(* Logix 5000 AddOnInstructionDefinition export AKD_Shutdown; software revision 26.01 *)

TYPE AKD_Status :   // All connections to the drive ethernet module are established and data is successfully transferring.
STRUCT
   Profile_In_Progress : BOOL;   // Profile Move In Progress
   Block_In_Execution : BOOL;   // Block In Execution
   On_Target_Position : BOOL;   // On Target Position (1=Current Position Equals Last Target Position)
   General_Fault : BOOL;   // General Fault
   Current_Direction : BOOL;   // Current Motor Direction (0=Reverse, 1=Forward)
   Home_Level : BOOL;   // Level of Home Input
   Reg_Level : BOOL;   // Level of Registration Input
   Enable : BOOL;   // State of Enable Output
   Fault_Input_Fault : BOOL;   // Fault Input Active
   Fwd_Limit : BOOL;   // Forward Input Active
   Rev_Limit : BOOL;   // Reverse Input Active
   Positive_Limit : BOOL;   // Positive Software Limit Exceeded
   Negative_Limit : BOOL;   // Negative Software Limit Exceeded
   FE_Fault : BOOL;   // Following Error Fault
   Block_Fault : BOOL;   // Block Execution Fault
   Load_Complete : BOOL;   // Command Message Successfully Loaded
END_STRUCT
END_TYPE

TYPE AKD_Control :   // Send Explicit Message
STRUCT
   Load_Data_Start_Profile : BOOL;   // Load Command Data / Start Profile Move
   Start_Block : BOOL;   // Execute Command block or block chain
   Incremental : BOOL;   // Incremental Position (0=Absolute, 1=Incremental)
   Direction : BOOL;   // Direction in Velocity Mode (0=Reverse, 1=Forward)
   Smooth_Stop : BOOL;   // Smooth / Controlled Stop w/ Deceleration
   Hard_Stop : BOOL;   // Hard / Immediate Stop
   Reg_Arm : BOOL;   // Arm the Registration Input
   Enable : BOOL;   // Enable Output
END_STRUCT
END_TYPE

TYPE AKD_Axis :   // Axis Data:
STRUCT
   Control : AKD_Control;   // Control bits to send to the drive
   Status : AKD_Status;   // Status bits received from the drive
   Input : AB:ETHERNET_MODULE_SINT_64Bytes:I:0;   // Data from the drive
   Output : AB:ETHERNET_MODULE_SINT_64Bytes:O:0;   // Data to the drive
   ResponseMsgType : SINT;   // Response type contained in latest IO response from drive. Used to check for errors
   CommandTimeout : INT;   // Time to allow for command response from drive. Dependent on scan rate and communicaiton rate
   PositionFeedback : DINT;   // Actual Position Value
   VelocityFeedback : DINT;   // Actual Velocity Value
END_STRUCT
END_TYPE

ADD_ON_INSTRUCTION AKD_Shutdown   (* revision 4.0, ExecutePrescan, ExecuteEnableInFalse *)
// Motion Hard Stop
// Revision note:
// There was a race with the Axis.Control.Hardstop bit.  I removed it from EnableInFalse and did the reset in the logic
VAR_OUTPUT
   DN : BOOL; {access Read Only, visible}   // Command Successful
   ER : BOOL; {access Read Only, visible}   // Error
END_VAR
VAR_IN_OUT
   Axis : AKD_Axis; {required}
END_VAR
VAR
   Command_Timeout : TIMER := (PRE := 2000);   // Timeout Timer
   Step : DINT; {access None}
END_VAR

ROUTINE EnableInFalse   (* ladder *)
// Enable In False
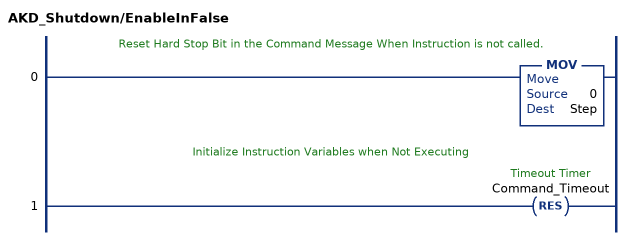
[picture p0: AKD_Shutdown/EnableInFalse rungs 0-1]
   // Reset Hard Stop Bit in the Command Message When Instruction is not called.
   0: MOV(0,Step);
   // Initialize Instruction Variables when Not Executing
   1: RES(Command_Timeout);
END_ROUTINE

ROUTINE Logic   (* ladder *)
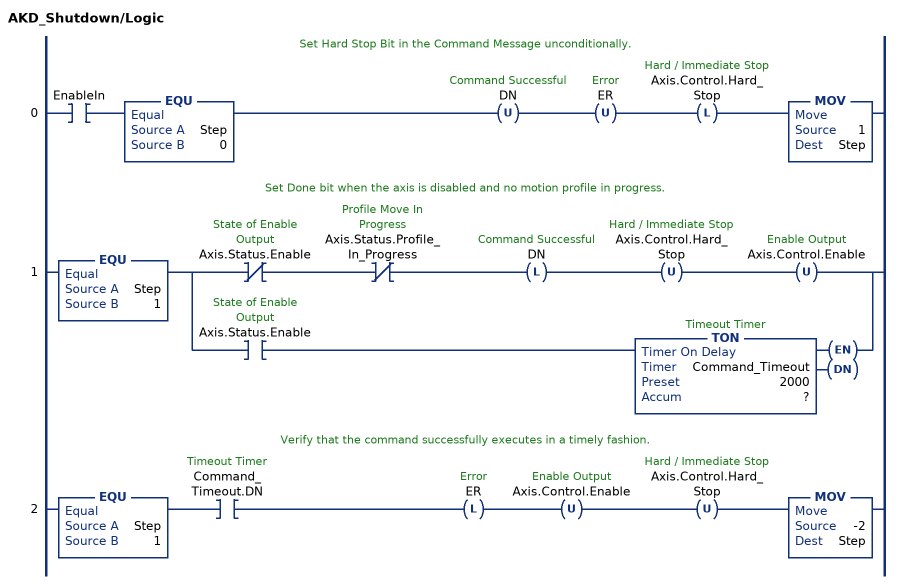
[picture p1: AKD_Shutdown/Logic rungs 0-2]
   // Set Hard Stop Bit in the Command Message unconditionally.
   0: XIC(EnableIn)EQU(Step,0)OTU(DN)OTU(ER)OTL(Axis.Control.Hard_Stop)MOV(1,Step);
   // Set Done bit when the axis is disabled and no motion profile in progress.
   1: EQU(Step,1)[XIO(Axis.Status.Enable) XIO(Axis.Status.Profile_In_Progress) OTL(DN) OTU(Axis.Control.Hard_Stop) OTU(Axis.Control.Enable) ,XIC(Axis.Status.Enable) TON(Command_Timeout,?,?) ];
   // Verify that the command successfully executes in a timely fashion.
   2: EQU(Step,1)XIC(Command_Timeout.DN)OTL(ER)OTU(Axis.Control.Enable)OTU(Axis.Control.Hard_Stop)MOV(-2,Step);
END_ROUTINE

ROUTINE Prescan   (* ladder *)
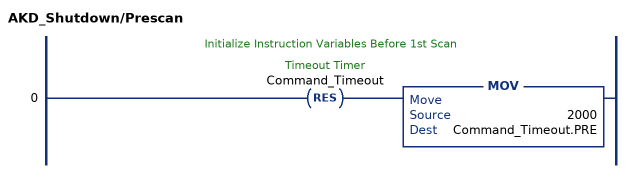
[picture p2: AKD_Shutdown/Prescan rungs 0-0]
   // Initialize Instruction Variables Before 1st Scan
   0: RES(Command_Timeout)MOV(2000,Command_Timeout.PRE);
END_ROUTINE
END_ADD_ON_INSTRUCTION
